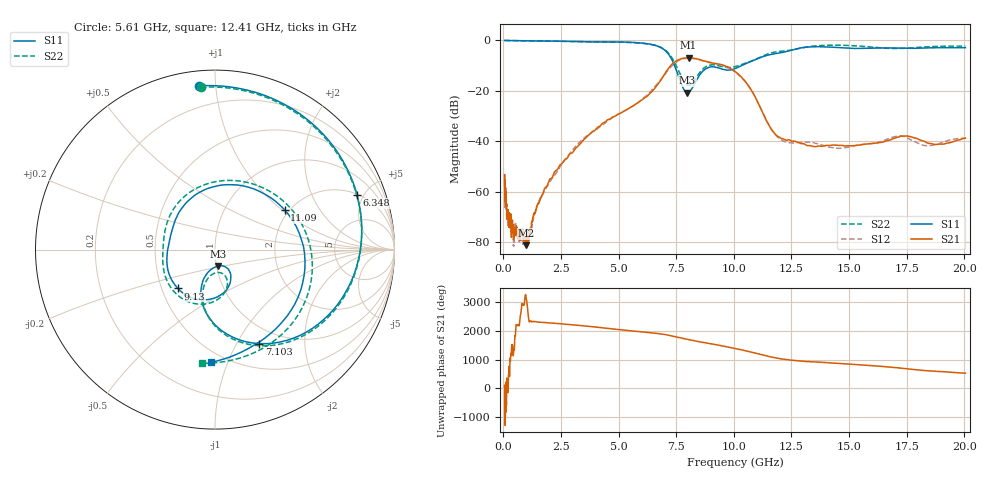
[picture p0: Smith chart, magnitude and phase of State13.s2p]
# Hz S DB R 50
!freq MagS11 AngS11 MagS21 AngS21 MagS12 AngS12 MagS22 AngS22
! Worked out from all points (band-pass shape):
!   1601 points, 50 MHz to 20.05 GHz, reference 50 ohm
!   highest |S21| = -6.87 dB at 8.038 GHz (marker M1); lowest = -81.3 dB at 975.3 MHz (marker M2)
!   |S21| within 3 dB of the highest: 7.267 GHz to 9.563 GHz (2.296 GHz wide, 27.3 % of centre)
!   lowest |S11| = -20.6 dB at 7.978 GHz (marker M3), VSWR 1.20, Z = 50.9 - j9.36 ohm
!   |S11| at or under -10 dB: 7.429 GHz to 10.33 GHz (2.9 GHz wide, 32.7 % of centre)
!   |S22| runs from -17.8 to 0.0 dB; largest |S21 - S12| = 0.029
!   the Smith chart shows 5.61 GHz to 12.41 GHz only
!   S11 on the Smith chart (normalised r, x): 5.61 GHz: 0.08, +0.90; 6.348 GHz: 2.07, +4.47; 7.103 GHz: 0.79, -1.24; 9.13 GHz: 0.60, -0.29; 11.09 GHz: 1.89, +1.05; 12.41 GHz: 0.42, -0.87
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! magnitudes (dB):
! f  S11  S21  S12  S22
! 50 MHz  0.0  -53.2  -53.7  0.0
! 55.95 MHz  0.0  -55.5  -53.1  0.0
! 59.63 MHz  0.0  -57.6  -65.0  0.0
! 70.84 MHz  0.0  -58.5  -56.7  0.0
! 135.9 MHz  0.0  -65.7  -68.3  0.0
! 369.6 MHz  0.0  -74.5  -72.5  0.0
! 445.8 MHz  0.0  -78.8  -81.4  -0.1
! 517.8 MHz  -0.1  -76.3  -72.7  -0.1
! 975.3 MHz  -0.1  -81.3  -77.6  -0.1
! 1.005 GHz  -0.1  -79.8  -79.7  -0.1
! 2.722 GHz  -0.3  -47.0  -46.8  -0.4
! 5.61 GHz  -0.8  -26.1  -26.1  -0.8
! 6.348 GHz  -1.4  -21.1  -20.5  -1.5
! 7.103 GHz  -4.8  -11.7  -12.3  -4.4
! 7.402 GHz  -9.4  -8.8  -9.3  -8.3
! 7.978 GHz  -20.6  -6.9  -7.1  -17.7
! 8.038 GHz  -20.5  -6.9  -7.1  -17.8
! 9.13 GHz  -10.5  -9.1  -8.9  -9.7
! 10.22 GHz  -10.5  -13.5  -13.7  -9.9
! 11.09 GHz  -7.0  -25.5  -25.5  -6.8
! 12.41 GHz  -4.0  -39.5  -40.6  -3.9
! 20.05 GHz  -2.9  -38.8  -38.7  -2.2
